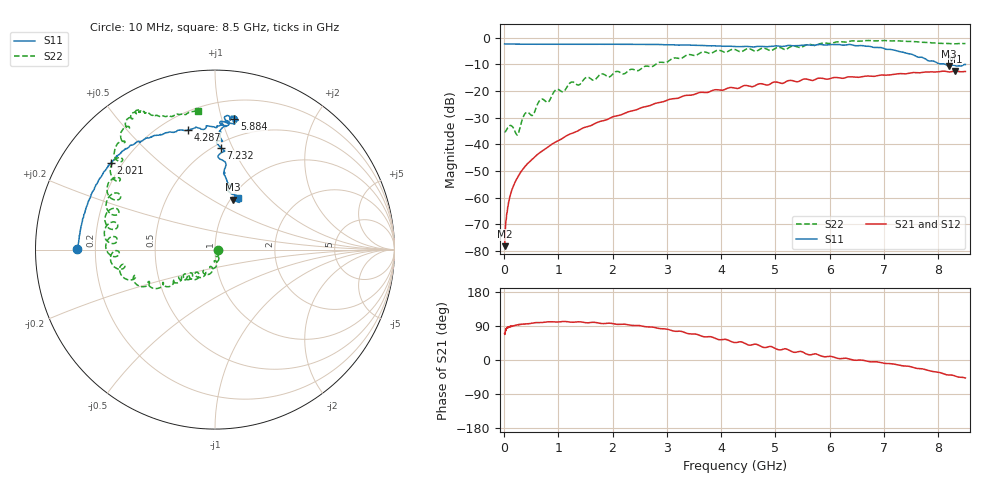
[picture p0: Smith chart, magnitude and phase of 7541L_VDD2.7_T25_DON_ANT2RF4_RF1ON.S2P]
!Agilent Technologies,E5071C,MY46417908,A.11.23
!Date: Wed Dec 09 17:17:24 2020
!Data & Calibration Information:
!Freq	S11:SOLT2(ON)	S21:SOLT2(ON)	S12:SOLT2(ON)	S22:SOLT2(ON)
!PortZ  Port1:50+j0  Port2:50+j0
!Above PortZ is port z conversion or system Z0 setting when saving the data.
!When reading, reference impedance value at option line is always used.
# Hz S dB R 50
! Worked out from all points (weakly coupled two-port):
!   1601 points, 10 MHz to 8.5 GHz, reference 50 ohm
!   highest |S21| = -12.49 dB at 8.304 GHz (marker M1); lowest = -78.1 dB at 10 MHz (marker M2)
!   lowest |S11| = -10.6 dB at 8.198 GHz (marker M3), VSWR 1.84, Z = 51.3 + j31.2 ohm
!   |S11| at or under -10 dB: 8.133 GHz to end of sweep
!   |S22| runs from -36.5 to -1.0 dB; largest |S21 - S12| = 0.0023
!   S11 on the Smith chart (normalised r, x): 10 MHz: 0.13, +0.00; 2.021 GHz: 0.16, +0.35; 4.287 GHz: 0.30, +0.75; 5.884 GHz: 0.35, +1.10; 7.232 GHz: 0.54, +0.90; 8.5 GHz: 1.07, +0.68
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1e7  -2.30 179.7  -78.13 69.9  -79.26 71.5  -35.32 -3.9
6.836875e7  -2.36 178.5  -63.29 85.7  -63.56 84.5  -33.69 -20.9
1.16125e8  -2.36 177.6  -59.02 88.3  -58.97 88.3  -32.91 -41.8
2.43475e8  -2.39 174.9  -52.55 92.8  -52.50 92.5  -36.46 -55.8
3.28375e8  -2.40 173.1  -49.77 94.5  -49.70 94.3  -31.10 -45.6
4.079688e8  -2.42 171.6  -47.80 95.4  -47.76 95.4  -28.00 -68.5
5.353188e8  -2.42 168.9  -45.28 97.1  -45.27 97.3  -28.97 -71.9
6.732812e8  -2.44 166.2  -42.84 98.9  -42.81 98.9  -23.18 -80.5
8.059375e8  -2.44 163.5  -41.01 100.7  -41.02 100.7  -24.20 -89.2
1.426769e9  -2.44 151.3  -34.10 100.4  -34.11 100.3  -16.76 -111.2
2.021069e9  -2.44 140.4  -29.52 95.2  -29.52 95.3  -13.22 -130.5
2.843538e9  -2.52 129.1  -24.33 83.4  -24.34 83.4  -9.33 -143.0
3.602331e9  -2.85 118.5  -20.52 65.1  -20.52 65.0  -5.81 -160.8
4.255e9  -3.31 103.9  -18.88 46.0  -18.88 46.0  -4.40 175.2
4.286838e9  -3.31 102.8  -19.00 46.3  -19.01 46.3  -4.66 173.1
5.671769e9  -2.82 80.5  -16.01 14.4  -15.96 14.3  -2.62 136.0
5.884019e9  -2.67 81.6  -15.26 9.0  -15.20 9.2  -1.92 132.8
7.088538e9  -4.34 87.4  -13.95 -9.3  -14.00 -9.4  -1.15 118.5
7.231806e9  -4.90 86.8  -13.57 -12.1  -13.57 -12.0  -1.14 118.3
8.197544e9  -10.61 70.5  -12.82 -39.6  -12.86 -39.6  -2.17 105.0
8.303669e9  -10.36 67.1  -12.49 -41.8  -12.50 -41.6  -2.26 102.6
8.5e9  -10.01 66.0  -12.64 -47.5  -12.72 -47.3  -2.17 97.1
